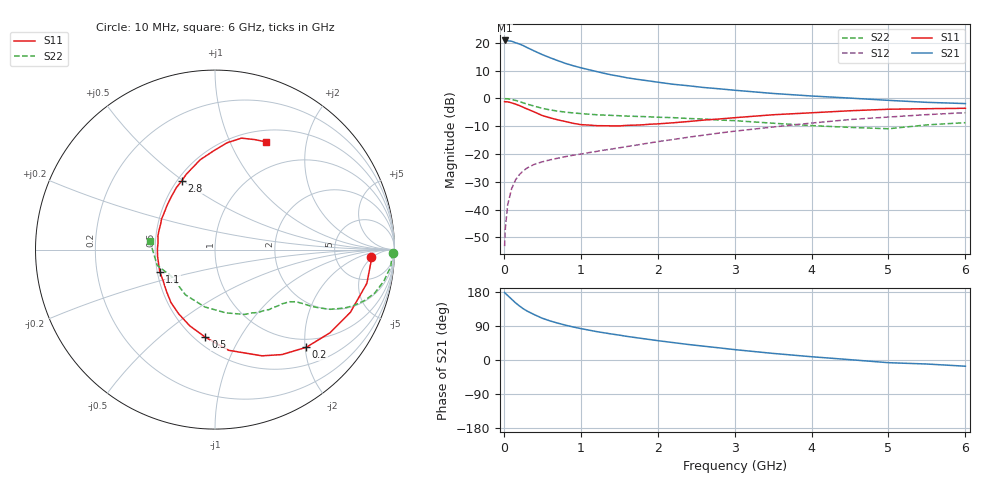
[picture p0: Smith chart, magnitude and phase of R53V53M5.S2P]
! SIEMENS Small Signal Semiconductors
! BFR183
! Si NPN RF Bipolar Junction Transistor in SOT23
! VCE = 3.5 V  IC = 3.5 mA
! Common Emitter S-Parameters:  May  1996
# GHz  S  MA  R  50
!  f  S11  S21  S12  S22
! GHz  MAG  ANG  MAG  ANG  MAG  ANG  MAG  ANG
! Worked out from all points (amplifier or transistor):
!   36 points, 10 MHz to 6 GHz, reference 50 ohm
!   highest |S21| = 20.8 dB at 10 MHz (marker M1)
!   |S21| within 3 dB of that: start of sweep to 336 MHz
!   unconditionally stable (mu >= 1): 1.183 GHz to 2.706 GHz
!   at 250 MHz: K = 0.33, MSG = 22.6 dB, |S12| = -26.1 dB
!   at 1.4 GHz: K = 1.06, MAG = 11.9 dB, |S12| = -18.2 dB
!   at 6 GHz: K = 0.89, MSG = 1.6 dB, |S12| = -5.1 dB
!   S11 on the Smith chart (normalised r, x): 10 MHz: 13, -4; 200 MHz: 0.83, -2.02; 500 MHz: 0.56, -0.73; 1.1 GHz: 0.52, -0.14; 2.8 GHz: 0.53, +0.50; 6 GHz: 0.64, +1.38
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0.01  0.8708 -2.6  11.01 178.2  0.0022 89.7  0.9928 -1.1
0.02  0.8711 -4.9  10.9 175.8  0.0047 90.9  0.9863 -2.2
0.05  0.8668 -12.5  10.86 170.2  0.0122 83.9  0.9841 -5.5
0.1  0.8314 -24.8  10.68 160.7  0.0235 77.0  0.9567 -10.6
0.15  0.7901 -36.0  10.03 151.2  0.0338 71.2  0.9225 -15.2
0.2  0.7446 -47.0  9.543 143.1  0.0423 66.7  0.8807 -18.8
0.25  0.6936 -57.5  8.931 135.6  0.0495 62.1  0.8327 -22.0
0.3  0.6473 -66.1  8.226 129.4  0.0558 59.4  0.7912 -24.3
0.4  0.5666 -82.2  7.082 119.3  0.0656 55.0  0.7228 -27.4
0.5  0.4915 -96.2  6.123 110.2  0.0723 52.3  0.6631 -29.3
0.6  0.4478 -108.2  5.393 103.2  0.0785 51.2  0.6206 -30.5
0.7  0.4113 -119.4  4.782 97.3  0.0839 51.0  0.5906 -31.2
0.8  0.3838 -129.7  4.264 92.0  0.0896 50.6  0.5663 -31.8
0.9  0.357 -139.1  3.872 87.2  0.095 51.1  0.548 -32.4
1.1  0.3315 -158.0  3.292 79.1  0.1055 52.7  0.5204 -34.0
1.6  0.3272 166.4  2.349 62.3  0.1362 55.2  0.4806 -38.9
2.2  0.3641 137.0  1.795 46.0  0.1822 55.9  0.4507 -47.8
2.8  0.4261 115.6  1.487 32.0  0.2379 53.4  0.408 -59.9
3.5  0.5077 99.3  1.226 17.4  0.3058 47.2  0.3576 -80.3
4.5  0.5991 83.5  1.012 0.9  0.4167 35.6  0.301 -123.2
5.5  0.652 70.0  0.849 -10.6  0.5104 22.4  0.3338 -164.7
6  0.664 64.6  0.807 -16.4  0.553 13.9  0.3663 172.3
